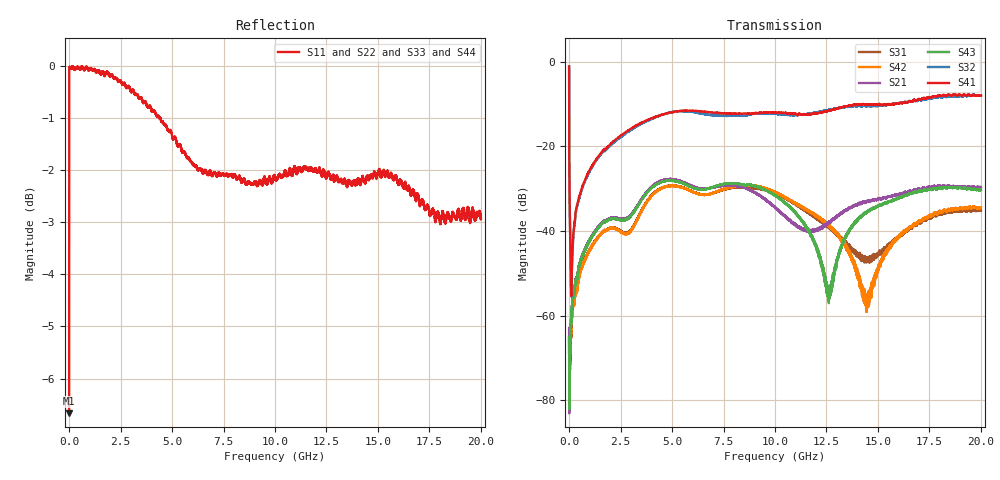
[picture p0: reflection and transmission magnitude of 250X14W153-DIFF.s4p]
!{250X14W153}
!Johanson Technology Inc.
!www.johansontechnology.com
!Test Board Conditions:
!Substrate Type  RO4350B
!Substrate Thickness  10 mil
!Substrate Dk  3.66
!TL Type: GCPW
!TL Trace Width  20 mil
!TL Gap  15 mil
!PART MODE DIFFERENTIAL
!DUT TOPOLOGY	DIFFERENTIAL 4-PORT
!Mounting Pad LxW  20x35 mil
# MHz S  dB  R 50
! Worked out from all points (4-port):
!   20001 points, 300 kHz to 20 GHz, reference 50 ohm
!   strongest paths, dB at 300 kHz, 5 GHz, 10 GHz, 15 GHz, 20 GHz:
!     S41: -1.1, -11.9, -12.0, -10.1, -8.0
!     S32: -1.1, -11.9, -12.3, -10.4, -7.9
!     S43: -65.2, -28.1, -31.6, -34.1, -30.3
!     S21: -62.9, -27.8, -34.4, -32.5, -29.7
!     S42: -65.6, -29.4, -30.8, -48.7, -34.4
!     S31: -68.7, -29.3, -31.1, -45.5, -35.1
!   lowest |S11| = -6.7 dB at 300 kHz (marker M1), VSWR 2.73, Z = 23.7 - j24.6 ohm
!   |S11| at or under -10 dB: nowhere
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0.3  -6.67 -118.4  -65.38 55.0  -64.98 30.8  -1.11 -27.6
     -62.88 46.2  -6.63 -119.1  -1.10 -27.4  -65.58 32.0
     -68.72 20.2  -1.07 -27.6  -6.68 -118.3  -63.91 41.1
     -1.11 -27.6  -65.61 63.1  -65.23 36.3  -6.66 -118.3
146.298  -0.03 178.7  -58.01 81.4  -59.31 78.4  -46.77 65.9
         -56.97 77.2  -0.05 178.9  -47.14 63.8  -59.23 76.6
         -59.70 81.8  -47.23 62.9  0.01 178.8  -57.66 80.6
         -46.82 65.5  -59.50 78.0  -57.59 82.3  -0.03 178.9
4620.231  -1.12 144.6  -27.88 37.4  -29.60 30.0  -12.38 34.4
          -27.91 37.5  -1.13 147.4  -12.40 35.1  -29.66 31.0
          -29.56 30.0  -12.38 35.2  -1.08 145.6  -28.24 37.5
          -12.38 34.5  -29.66 31.2  -28.25 37.2  -1.09 145.7
10073.15  -2.18 121.1  -34.68 -43.5  -31.26 -75.7  -12.00 -8.0
          -34.68 -43.2  -2.18 121.2  -12.32 -7.4  -30.96 -78.7
          -31.31 -75.7  -12.31 -7.5  -2.04 118.1  -31.78 -53.9
          -12.03 -8.0  -30.90 -78.6  -31.77 -53.6  -2.42 119.7
12613.11  -2.09 109.9  -38.15 11.6  -39.06 -107.4  -11.48 -10.3
          -37.78 13.3  -2.18 116.2  -11.33 -10.4  -38.48 -119.2
          -39.10 -107.5  -11.41 -10.0  -1.91 109.0  -54.10 -16.6
          -11.51 -10.0  -38.45 -119.2  -54.17 -14.3  -2.17 115.4
14456.08  -2.13 95.8  -33.07 9.6  -46.77 -68.8  -10.06 -19.5
          -33.03 9.1  -2.17 100.0  -10.50 -20.8  -56.24 -64.9
          -46.47 -69.0  -10.46 -20.5  -2.26 92.5  -35.50 33.1
          -10.03 -19.5  -56.51 -71.4  -35.60 33.1  -2.53 95.2
20000  -2.93 64.1  -29.73 -37.5  -35.03 -75.0  -7.99 -46.9
       -29.65 -37.8  -3.03 68.8  -7.93 -47.3  -34.36 -68.7
       -35.14 -74.3  -7.92 -46.2  -2.98 60.9  -30.21 -32.3
       -7.98 -46.4  -34.38 -68.6  -30.30 -33.0  -2.96 64.3
